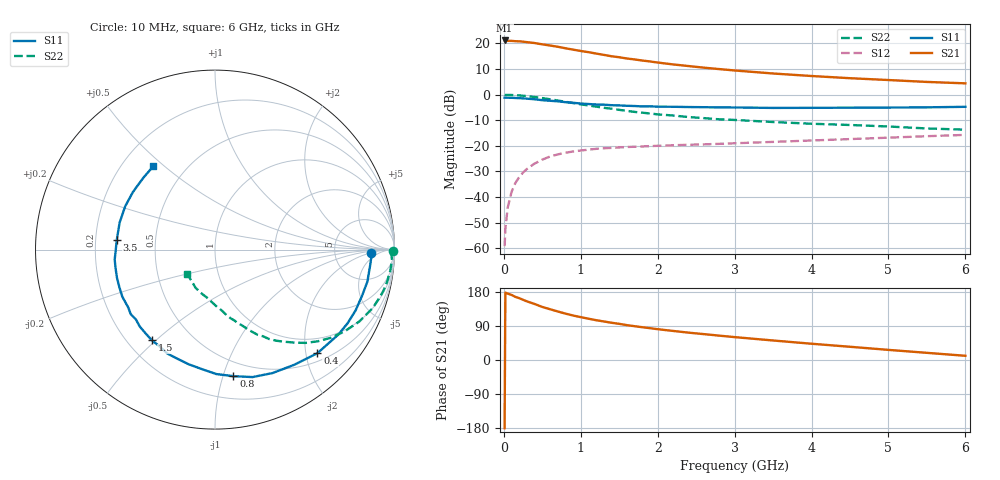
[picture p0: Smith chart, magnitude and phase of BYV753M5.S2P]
! SIEMENS Small Signal Semiconductors
! BFY420
! Si NPN RF SIEGET Grounded Emitter Transistor in MICRO-X
! VCE = 0.75 V  IC = 3.5 mA
! Common Emitter S-Parameters:  October  1996
# GHz  S  MA  R  50
!  f  S11  S21  S12  S22
! GHz  MAG  ANG  MAG  ANG  MAG  ANG  MAG  ANG
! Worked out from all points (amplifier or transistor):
!   36 points, 10 MHz to 6 GHz, reference 50 ohm
!   highest |S21| = 21.1 dB at 10 MHz (marker M1)
!   |S21| within 3 dB of that: start of sweep to 792.7 MHz
!   unconditionally stable (mu >= 1): 3.37 GHz to end of sweep
!   at 250 MHz: K = 0.08, MSG = 25.5 dB, |S12| = -30.4 dB
!   at 1.4 GHz: K = 0.45, MSG = 17.9 dB, |S12| = -20.8 dB
!   at 6 GHz: K = 1.21, MAG = 7.3 dB, |S12| = -15.7 dB
!   S11 on the Smith chart (normalised r, x): 10 MHz: 14, -2; 400 MHz: 0.66, -2.23; 800 MHz: 0.38, -1.08; 1.5 GHz: 0.30, -0.49; 3.5 GHz: 0.29, +0.05; 6 GHz: 0.33, +0.46
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0.01  0.8701 -1.4  11.41 -179.9  0.0011 90.3  0.9894 -0.6
0.02  0.8724 -2.6  11.39 177.9  0.0024 92.7  0.983 -1.3
0.05  0.8687 -6.0  11.21 175.2  0.0062 87.2  0.988 -3.4
0.1  0.8675 -11.9  11.19 171.8  0.0126 83.0  0.9834 -7.0
0.15  0.8589 -17.3  11.03 166.6  0.0189 80.0  0.9755 -10.5
0.2  0.8535 -23.4  10.98 163.2  0.0245 77.3  0.966 -13.8
0.25  0.845 -29.1  10.82 158.8  0.0302 73.5  0.95 -17.3
0.4  0.8117 -45.3  10.16 147.8  0.0451 65.1  0.8983 -26.5
0.5  0.7792 -55.4  9.58 140.0  0.0539 59.7  0.8552 -32.1
0.6  0.7589 -65.0  9.101 134.0  0.0619 55.3  0.8121 -37.2
0.8  0.7126 -81.7  8.042 122.5  0.0732 47.1  0.7251 -45.8
0.9  0.6934 -89.4  7.556 117.4  0.0776 44.3  0.684 -49.3
1.1  0.6554 -103.0  6.745 109.0  0.0843 39.1  0.6135 -55.9
1.3  0.637 -114.7  5.97 101.7  0.0897 35.0  0.5533 -60.9
1.5  0.6158 -124.8  5.367 95.4  0.0931 31.8  0.5044 -65.5
1.8  0.588 -138.5  4.625 86.5  0.0974 28.4  0.4438 -70.9
2.2  0.5793 -153.1  3.886 76.7  0.1027 25.3  0.3909 -77.4
2.8  0.5635 -169.6  3.152 64.3  0.1094 22.5  0.3296 -85.6
3.5  0.5499 174.2  2.585 51.5  0.1195 20.4  0.2919 -93.7
4.5  0.5555 154.3  2.092 34.9  0.1356 16.7  0.2554 -107.1
5.5  0.5651 135.1  1.769 18.9  0.1543 12.0  0.2185 -126.5
6  0.5779 126.5  1.66 11.1  0.1637 9.3  0.2069 -138.6
